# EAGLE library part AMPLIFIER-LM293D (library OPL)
Low Power Dual Voltage Comparators
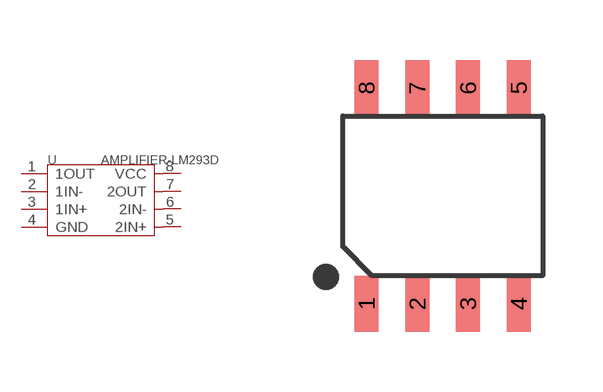
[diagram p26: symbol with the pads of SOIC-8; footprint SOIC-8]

Designator prefix U

## AMPLIFIER-LM293D-310020016  [SOIC-8]
1  1OUT  out
2  1IN-  in
3  1IN+  in
4  GND  sup
5  2IN+  in
6  2IN-  in
7  2OUT  out
8  VCC  sup

## Footprint SOIC-8 (pad centres in mm)
smd 0.6 x 1.4: 1 -1.905,-2.7; 2 -0.635,-2.7; 3 0.635,-2.7; 4 1.905,-2.7; 5 1.905,2.7; 6 0.635,2.7; 7 -0.635,2.7; 8 -1.905,2.7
